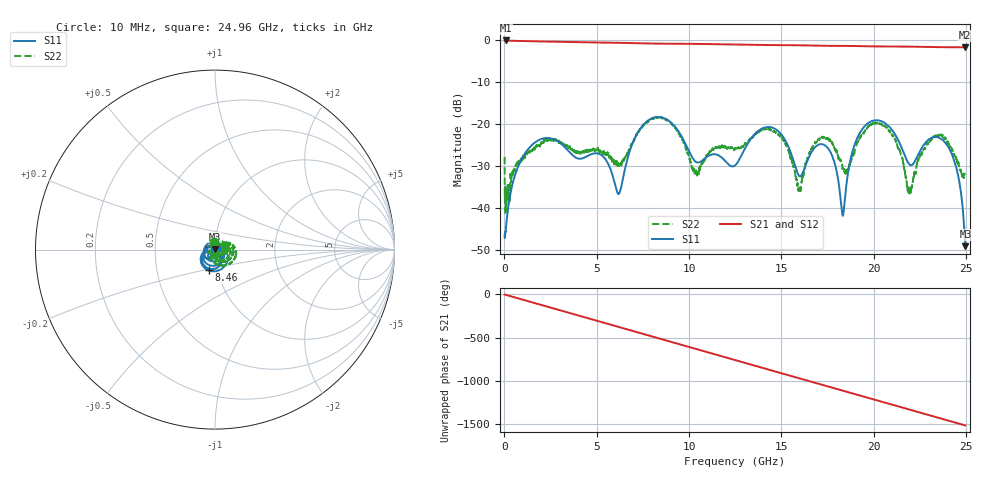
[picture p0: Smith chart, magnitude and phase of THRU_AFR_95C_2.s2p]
!Keysight Technologies,M9372A,MY54321388,A.12.55.09
!Automatic Fixture Removal (AFR)
!Date: Wednesday, May 22, 2019 8:34:27 AM
!S2P File: Measurements: S11,S21,S12,S22:
# MHz S  RI  R 50
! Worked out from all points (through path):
!   2496 points, 10 MHz to 24.96 GHz, reference 50 ohm
!   highest |S21| = -0.03 dB at 70 MHz (marker M1); lowest = -1.7 dB at 24.94 GHz (marker M2)
!   group delay of S21, straight-line fit = 169 ps
!   lowest |S11| = -49.1 dB at 24.96 GHz (marker M3), VSWR 1.01, Z = 50.2 + j0.29 ohm
!   |S11| at or under -10 dB: start of sweep to end of sweep
!   |S22| runs from -41.6 to -18.3 dB; largest |S21 - S12| = 1.4e-15
!   S11 on the Smith chart (normalised r, x): 10 MHz: 1.01, +0.00; 8.46 GHz: 0.91, -0.21; 24.96 GHz: 1.00, +0.01
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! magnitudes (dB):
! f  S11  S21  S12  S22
! 10 MHz  -46.4  -0.1  -0.1  -27.8
! 70 MHz  -45.7  0.0  0.0  -39.4
! 1.53 GHz  -24.8  -0.2  -0.2  -25.9
! 4.17 GHz  -28.2  -0.4  -0.4  -26.7
! 6.19 GHz  -36.7  -0.6  -0.6  -29.5
! 7.14 GHz  -22.6  -0.7  -0.7  -22.5
! 8.33 GHz  -18.3  -0.8  -0.8  -18.3
! 8.46 GHz  -18.4  -0.8  -0.8  -18.3
! 10.39 GHz  -29.1  -0.9  -0.9  -32.3
! 12.49 GHz  -29.9  -1.0  -1.0  -25.8
! 14.39 GHz  -20.7  -1.1  -1.1  -21.2
! 15.96 GHz  -32.4  -1.2  -1.2  -36.1
! 16.65 GHz  -26.5  -1.2  -1.2  -25.7
! 17.64 GHz  -26.6  -1.3  -1.3  -23.9
! 18.32 GHz  -41.9  -1.3  -1.3  -30.3
! 19.23 GHz  -22.2  -1.4  -1.4  -23.3
! 20.81 GHz  -20.5  -1.5  -1.5  -21.5
! 21.94 GHz  -29.7  -1.5  -1.5  -35.4
! 23.95 GHz  -24.9  -1.6  -1.6  -24.0
! 24.57 GHz  -32.3  -1.7  -1.7  -29.6
! 24.94 GHz  -48.0  -1.7  -1.7  -32.1
! 24.96 GHz  -49.1  -1.7  -1.7  -32.1
